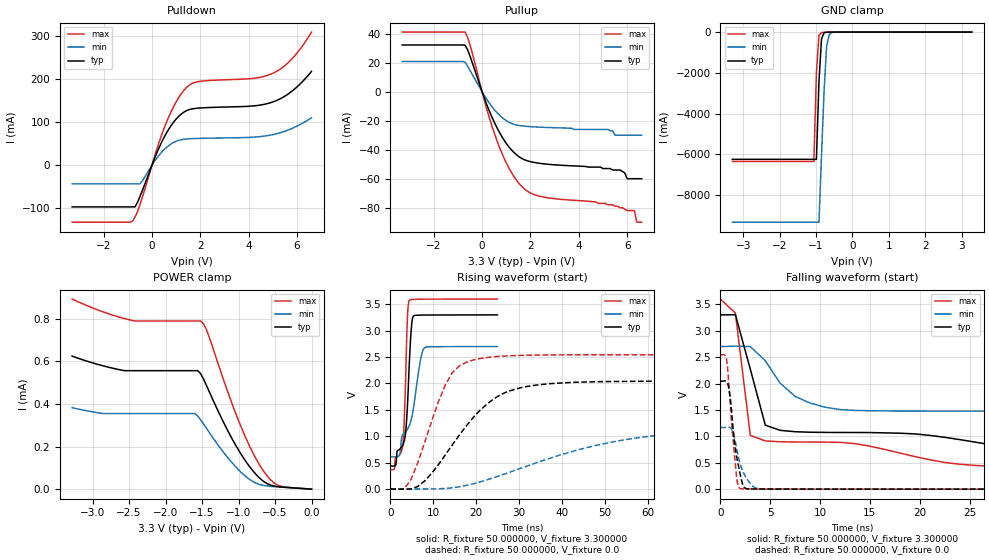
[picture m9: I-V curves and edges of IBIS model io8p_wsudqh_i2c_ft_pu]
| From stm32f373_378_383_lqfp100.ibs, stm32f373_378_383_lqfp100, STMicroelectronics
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|   Model io8p_wsudqh_i2c_ft_pu
[Model]  io8p_wsudqh_i2c_ft_pu
Model_type I/O
Polarity   Non-Inverting
Enable   Active-Low
Vinl =   0.990000V
Vinh =   2.310000V
Vmeas =  1.650000V
Cref =   30.000000pF
Rref =   100.000000M
Vref =   0.0V
C_comp   0.0F   0.0F   0.0F
[Temperature Range]   25.000000   0.140000k   -40.000000
[Pullup Reference]   3.300000V   2.700000V   3.600000V
[Pulldown Reference]   0.0V   0.0V   0.0V
[POWER Clamp Reference]   3.300000V   2.700000V   3.600000V
[GND Clamp Reference]   0.0V   0.0V   0.0V
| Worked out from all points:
|   slope of the pulldown table from 0 to 0.495 V, typ, clamps not added: 7.75 ohm
|   slope of the pullup table from 0 to 0.495 V, typ, clamps not added: 23.9 ohm
|   GND clamp passes 1 mA (typ) near -0.61 V on its own axis
|   rising waveform, R_fixture 50.000000, V_fixture 3.300000: 20-80 % time 1.17ns typ, 3.83ns min, 774ps max; typ from 0.435 V to 3.3 V
|   rising waveform, R_fixture 50.000000, V_fixture 0.0: 20-80 % time 12.2ns typ, 29.8ns min, 6.8ns max; typ from 0 V to 2.04 V
|   falling waveform, R_fixture 50.000000, V_fixture 3.300000: 20-80 % time 19.1ns typ, 55.7ns min, 1.33ns max; typ from 3.3 V to 0.435 V
|   falling waveform, R_fixture 50.000000, V_fixture 0.0: 20-80 % time 806ps typ, 1.08ns min, 654ps max; typ from 2.04 V to 0 V
[Pulldown]
|Voltage   I(typ)   I(min)   I(max)
-3.3V     -96.33mA   -43.01mA   -131.7mA
-800mV    -96.33mA   -43.01mA   -129.4mA
-700mV    -96.33mA   -43.01mA   -120mA
-500mV    -72.9mA    -43.01mA   -92.16mA
200mV     28.44mA    16.57mA    37.01mA
600mV     74.69mA    41.37mA    99.56mA
1V        107mA      55.62mA    146.8mA
1.4V      125.8mA    60.81mA    178.5mA
1.9V      132.3mA    62.32mA    193.7mA
5V        146.8mA    71.07mA    213.2mA
5.8V      172.1mA    85.55mA    247mA
6.6V      217.6mA    110.2mA    308.5mA
[Pullup]
|Voltage   I(typ)   I(min)   I(max)
-3.3V     32.23mA    20.82mA    41.12mA
-700mV    32.07mA    20.32mA    41.12mA
200mV     -9.092mA   -5.447mA   -12.2mA
700mV     -27.48mA   -15.83mA   -37.39mA
1.2V      -39.86mA   -21.7mA    -55.32mA
1.8V      -47.22mA   -23.81mA   -67.73mA
5.2V      -53mA      -26mA      -78mA
5.7V      -54mA      -30mA      -80mA
6V        -60mA      -30mA      -82mA
6.3V      -60mA      -30mA      -82mA
6.4V      -60mA      -30mA      -90mA
6.6V      -60mA      -30mA      -90mA
[GND_clamp]
|Voltage   I(typ)   I(min)   I(max)
-3.3V     -6.241A    -9.325A    -6.345A
-1.06V    -6.241A    -9.325A    -6.345A
-990mV    -6.241A    -9.325A    -2.007A
-920mV    -2.435A    -9.325A    -157.2mA
-850mV    -331.1mA   -6.034A    -23.1mA
-780mV    -36.12mA   -2.918A    -12.65mA
-710mV    -6.437mA   -709.1mA   -7.385mA
-640mV    -1.621mA   -128.1mA   -3.348mA
-570mV    -372.4uA   -25.26mA   -954.9uA
3.28V     0A         5.405nA    0A
[POWER_clamp]
|Voltage   I(typ)   I(min)   I(max)
-3.28V    623.9uA    382uA      891.7uA
-2.88V    580.8uA    355.8uA    834.6uA
-2.44V    555.9uA    354.7uA    789.9uA
-1.6V     555.9uA    354.7uA    788.9uA
-1.52V    542.1uA    325.9uA    788.9uA
-1.44V    486.9uA    285.5uA    748.6uA
-1.04V    206.7uA    105.3uA    356.5uA
-840mV    101.9uA    43.53uA    195.7uA
-680mV    42.68uA    18.98uA    96.33uA
-560mV    18.58uA    13.4uA     43.73uA
-440mV    10.88uA    10.3uA     15.86uA
0V        0A         6.245nA    0A
[Ramp]
| variable   typ   min   max
dV/dt_r  1.22654/12.15583n   0.69950/29.74812n   1.52650/6.74539n
dV/dt_f  1.71876/18.83155n   1.25324/55.61744n   1.94057/1.26340n
R_load = 50.000000
[Rising Waveform]
R_fixture= 50.000000
V_fixture= 3.300000
V_fixture_min= 2.700000
V_fixture_max= 3.600000
|time   V(typ)   V(min)   V(max)
0s        435.4mV    610mV      365.7mV
2.102ns   749mV      639mV      643.4mV
2.903ns   833.2mV    1.032V     827mV
3.253ns   915.1mV    1.061V     1.319V
3.654ns   1.145V     1.095V     2.354V
4.004ns   1.597V     1.136V     3.267V
4.404ns   2.343V     1.199V     3.569V
5.205ns   3.243V     1.44V      3.592V
7.908ns   3.297V     2.674V     3.598V
24.92ns   3.3V       2.7V       3.6V
[Rising Waveform]
R_fixture= 50.000000
V_fixture= 0.0
V_fixture_min= 0.0
V_fixture_max= 0.0
|time   V(typ)   V(min)   V(max)
0s        461.3uV    573.5uV    437.5uV
3.203ns   -553uV     192.7uV    1.446mV
4.805ns   588.6uV    9.087uV    176.9mV
11.21ns   464.9mV    4.479mV    1.659V
14.41ns   834.5mV    22.85mV    2.203V
20.82ns   1.488V     133.3mV    2.473V
28.83ns   1.886V     348.9mV    2.529V
56.06ns   2.04V      952.7mV    2.545V
92.89ns   2.045V     1.144V     2.545V
797.6ns   2.045V     1.167V     2.545V
[Falling Waveform]
R_fixture= 50.000000
V_fixture= 3.300000
V_fixture_min= 2.700000
V_fixture_max= 3.600000
|time   V(typ)   V(min)   V(max)
0s        3.3V       2.7V       3.6V
1.502ns   3.304V     2.708V     3.335V
3.003ns   2.272V     2.7V       1.018V
4.505ns   1.213V     2.433V     914.2mV
6.006ns   1.114V     2.006V     898.1mV
12.01ns   1.074V     1.507V     887.2mV
33.03ns   660.7mV    1.464V     401.6mV
78.08ns   447mV      782.7mV    367mV
123.1ns   437mV      646.6mV    365.8mV
747.7ns   435.4mV    610mV      365.7mV
[Falling Waveform]
R_fixture= 50.000000
V_fixture= 0.0
V_fixture_min= 0.0
V_fixture_max= 0.0
|time   V(typ)   V(min)   V(max)
0s        2.045V     1.167V     2.545V
600.6ps   2.037V     1.172V     2.476V
700.7ps   2.01V      1.175V     2.349V
1.001ns   1.71V      1.162V     1.574V
1.301ns   1.087V     1.053V     885.2mV
1.602ns   653.9mV    800.7mV    268.1mV
2.002ns   268mV      465.2mV    12.01mV
2.402ns   29mV       279.9mV    5.709mV
4.004ns   3.212mV    7.07mV     2.684mV
49.85ns   461.3uV    573.5uV    437.5uV
